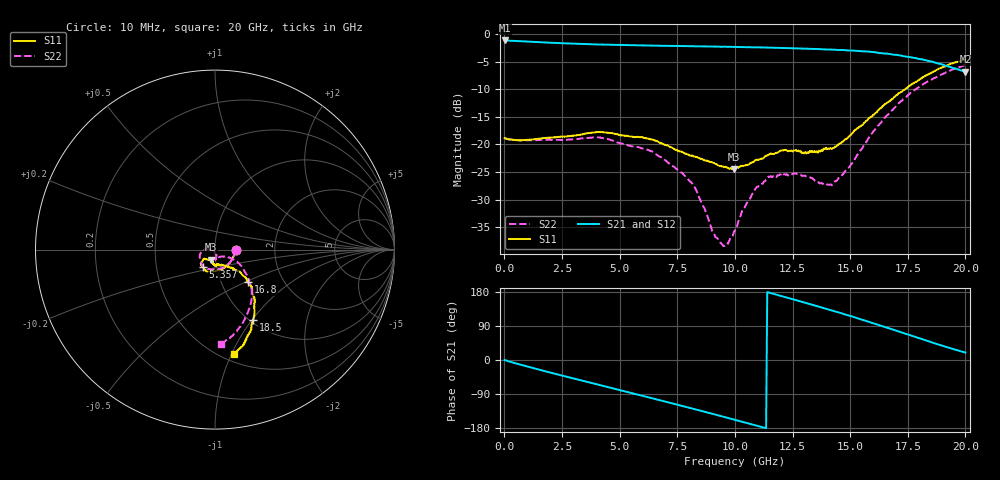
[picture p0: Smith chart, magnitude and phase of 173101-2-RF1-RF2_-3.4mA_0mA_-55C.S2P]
!  2-Port S-parameters saved by WinCal
! VAR MeasName=S-Parameters (CALIBRATED_DATA) read from VNA (N5242A)
! VAR MeasDate=2017-7-20 10:22:28
! VAR NAME=173101-2-RF1-RF2_-3.4mA_0mA_-55C
! VAR FILENAME=173101-2-RF1-RF2_-3.4mA_0mA_-55C.S2P
! VAR DATE=2017-7-20 10:22:28
! VAR PHYS_PORTS=1,2
# Hz S DB R 50
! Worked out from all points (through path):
!   401 points, 10 MHz to 20 GHz, reference 50 ohm
!   highest |S21| = -1.09 dB at 10 MHz (marker M1); lowest = -6.8 dB at 20 GHz (marker M2)
!   group delay of S21, straight-line fit = 46.6 ps
!   lowest |S11| = -24.5 dB at 9.955 GHz (marker M3), VSWR 1.13, Z = 47.7 - j5.35 ohm
!   |S11| at or under -10 dB: start of sweep to 17.37 GHz
!   |S22| runs from -38.5 to -5.6 dB; largest |S21 - S12| = 0.0074
!   S11 on the Smith chart (normalised r, x): 10 MHz: 1.26, -0.01; 5.357 GHz: 0.86, -0.17; 16.8 GHz: 1.34, -0.51; 18.5 GHz: 1.04, -1.01; 20 GHz: 0.57, -1.02
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1e7  -18.84 -1.9  -1.09 -0.0  -1.10 -0.1  -18.82 -1.8
1.50925e9  -18.95 -56.9  -1.41 -25.6  -1.42 -25.6  -19.19 -59.4
3.358325e9  -18.16 -98.5  -1.73 -54.3  -1.74 -54.3  -18.88 -108.2
5.357325e9  -18.46 -124.1  -1.94 -84.7  -1.96 -84.7  -20.17 -145.4
6.70665e9  -19.59 -136.3  -2.04 -105.6  -2.04 -105.6  -22.15 -167.9
8.2059e9  -22.15 -139.9  -2.15 -129.0  -2.16 -129.0  -27.51 174.6
9.055475e9  -23.34 -124.3  -2.19 -142.5  -2.19 -142.5  -35.90 -159.2
9.4053e9  -23.88 -119.7  -2.24 -148.1  -2.23 -148.3  -37.96 -134.4
9.6052e9  -24.03 -116.3  -2.23 -151.4  -2.24 -151.4  -38.09 -119.1
9.955025e9  -24.49 -110.4  -2.25 -157.0  -2.28 -157.2  -35.92 -93.8
1.0005e10  -24.28 -110.7  -2.27 -157.9  -2.28 -158.0  -35.61 -91.0
1.04048e10  -23.84 -103.9  -2.30 -164.4  -2.31 -164.5  -31.62 -78.0
1.085458e10  -22.99 -100.3  -2.35 -171.7  -2.37 -171.8  -28.31 -75.5
1.145428e10  -21.87 -97.3  -2.39 178.4  -2.42 178.3  -25.82 -80.7
1.255372e10  -21.08 -85.7  -2.51 159.7  -2.53 159.7  -25.23 -87.4
1.335332e10  -21.18 -79.7  -2.62 145.9  -2.60 145.8  -26.09 -85.1
1.430285e10  -20.62 -65.8  -2.78 129.0  -2.79 128.9  -26.91 -65.3
1.555222e10  -16.40 -45.1  -3.07 105.8  -3.08 105.5  -20.51 -28.8
1.670165e10  -12.09 -43.4  -3.54 83.2  -3.59 82.8  -14.30 -34.5
1.68016e10  -11.80 -44.1  -3.64 81.3  -3.64 81.4  -13.86 -36.2
1.850075e10  -7.05 -61.4  -4.89 47.4  -4.96 47.1  -8.27 -61.0
2e10  -4.54 -79.7  -6.78 19.7  -6.85 20.2  -5.56 -86.6
